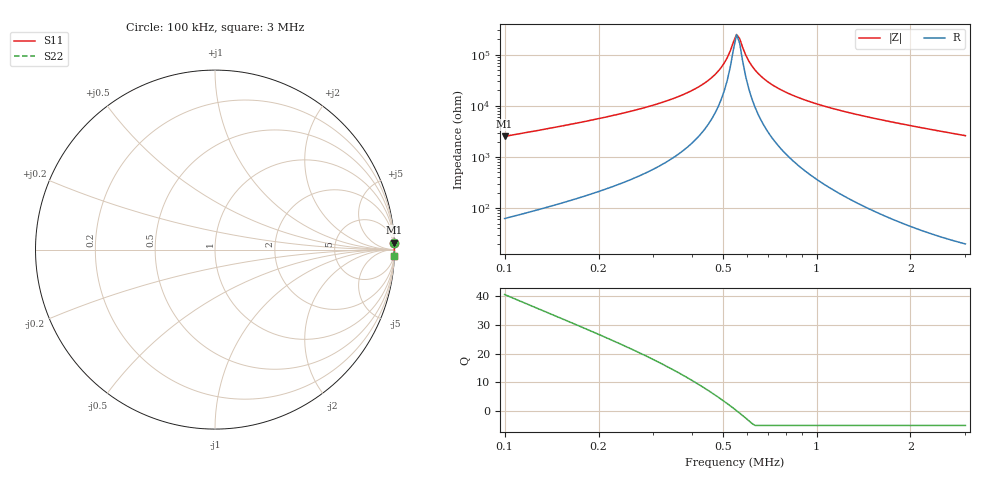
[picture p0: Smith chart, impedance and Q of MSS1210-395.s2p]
# MHz S MA R 50
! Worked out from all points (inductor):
!   150 points, 100 kHz to 3 MHz, reference 50 ohm
!   read as one part in series: L = 3.9 mH near 100 kHz
!   highest Q = 40.5 at 100 kHz (marker M1), where L = 4.03 mH
!   self-resonance near 554 kHz
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0.1  0.9982 2.3  0.03943 -86.3  0.03943 -86.3  0.9982 2.3
0.1690488  0.999 1.3  0.0219 -86.8  0.0219 -86.8  0.999 1.3
0.3590539  0.9995 0.4  0.006643 -85.4  0.006643 -85.4  0.9995 0.4
0.4409423  0.9996 0.2  0.003464 -82.4  0.003464 -82.4  0.9996 0.2
0.4721962  0.9996 0.1  0.002449 -79.8  0.002449 -79.8  0.9996 0.1
0.5056653  0.9996 0.1  0.001458 -73.4  0.001458 -73.4  0.9996 0.1
0.5292858  0.9996 0.0  0.0008321 -60.8  0.0008321 -60.8  0.9996 0.0
0.5540098  0.9996 0.0  0.0004006 -8.1  0.0004006 -8.1  0.9996 0.0
0.5668015  0.9996 -0.0  0.0004809 35.3  0.0004809 35.3  0.9996 -0.0
0.5798886  0.9996 -0.0  0.0007257 57.6  0.0007257 57.6  0.9996 -0.0
0.5932778  0.9996 -0.1  0.001023 67.9  0.001023 67.9  0.9996 -0.1
0.6209909  0.9996 -0.1  0.001664 76.9  0.001664 76.9  0.9996 -0.1
0.6499985  0.9996 -0.1  0.002326 80.8  0.002326 80.8  0.9996 -0.1
0.6960702  0.9996 -0.2  0.003339 83.7  0.003339 83.7  0.9996 -0.2
0.7454075  0.9996 -0.2  0.004372 85.2  0.004372 85.2  0.9996 -0.2
0.8745582  0.9997 -0.4  0.006878 86.9  0.006878 86.9  0.9997 -0.4
1.074016  0.9997 -0.6  0.01037 87.8  0.01037 87.8  0.9997 -0.6
1.289197  0.9996 -0.8  0.01384 88.1  0.01384 88.1  0.9996 -0.8
1.583221  0.9996 -1.0  0.01831 88.1  0.01831 88.1  0.9996 -1.0
2.035123  0.9994 -1.4  0.02483 88.0  0.02483 88.0  0.9994 -1.4
2.556974  0.9992 -1.8  0.03212 87.7  0.03212 87.7  0.9992 -1.8
3  0.999 -2.2  0.03818 87.4  0.03818 87.4  0.999 -2.2
